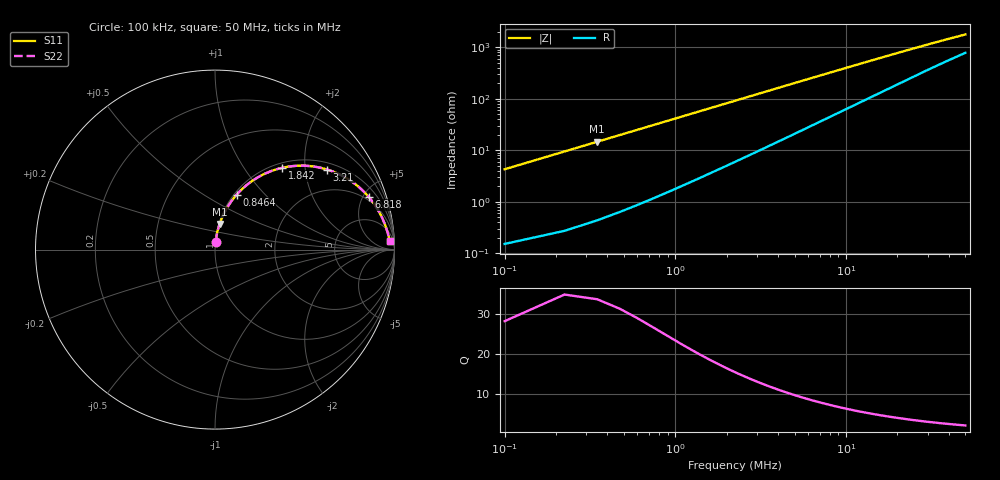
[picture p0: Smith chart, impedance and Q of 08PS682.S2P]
! Coilcraft 0805PS-682 Power Chip Inductor
! 5 February 2003
# MHZ S MA R 50
!Freq  MagS11  AngS11  MagS21  AngS21  MagS12  AngS12  MagS22  AngS22
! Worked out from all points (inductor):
!   403 points, 100 kHz to 50 MHz, reference 50 ohm
!   read as one part in series: L = 6.68 uH near 348.8 kHz
!   highest Q = 28.3 at 348.8 kHz (marker M1), where L = 6.71 uH
!   S11 on the Smith chart (normalised r, x): 100 kHz: 1.00, +0.09; 846.4 kHz: 1.03, +0.71; 1.842 MHz: 1.09, +1.52; 3.21 MHz: 1.21, +2.62; 6.818 MHz: 1.69, +5.48; 50 MHz: 17, +32
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0.1  0.04263 85.5  0.9976 -2.4  0.9976 -2.4  0.04263 85.5
0.2244  0.09436 83.0  0.9928 -5.4  0.9928 -5.4  0.09436 83.0
0.3488  0.1448 80.0  0.9852 -8.3  0.9852 -8.3  0.1448 80.0
0.4732  0.1938 77.0  0.9749 -11.2  0.9749 -11.2  0.1938 77.0
0.5976  0.2409 74.1  0.9623 -13.9  0.9623 -13.9  0.2409 74.1
0.8464  0.3289 68.5  0.9314 -19.2  0.9314 -19.2  0.3289 68.5
1.2196  0.4436 61.0  0.8756 -26.3  0.8756 -26.3  0.4436 61.0
1.4684  0.5084 56.5  0.8353 -30.5  0.8353 -30.5  0.5084 56.5
1.8416  0.5894 50.6  0.7744 -36.0  0.7744 -36.0  0.5894 50.6
2.4636  0.689 42.7  0.6793 -43.4  0.6793 -43.4  0.689 42.7
3.21  0.7676 35.5  0.583 -49.9  0.583 -49.9  0.7676 35.5
3.9564  0.8185 30.3  0.506 -54.6  0.506 -54.6  0.8185 30.3
4.7028  0.8527 26.3  0.4447 -58.0  0.4447 -58.0  0.8527 26.3
5.698  0.8829 22.3  0.3814 -61.3  0.3814 -61.3  0.8829 22.3
6.8176  0.9049 19.0  0.3279 -63.9  0.3279 -63.9  0.9049 19.0
8.4348  0.9245 15.6  0.272 -66.2  0.272 -66.2  0.9245 15.6
12.1668  0.9466 11.1  0.1951 -68.6  0.1951 -68.6  0.9466 11.1
16.7696  0.9581 8.1  0.145 -69.2  0.145 -69.2  0.9581 8.1
25.1044  0.9669 5.5  0.09994 -67.9  0.09994 -67.9  0.9669 5.5
33.4392  0.971 4.2  0.07712 -65.8  0.07712 -65.8  0.971 4.2
41.774  0.9733 3.3  0.06342 -63.4  0.06342 -63.4  0.9733 3.3
50  0.9749 2.8  0.05443 -61.1  0.05443 -61.1  0.9749 2.8
